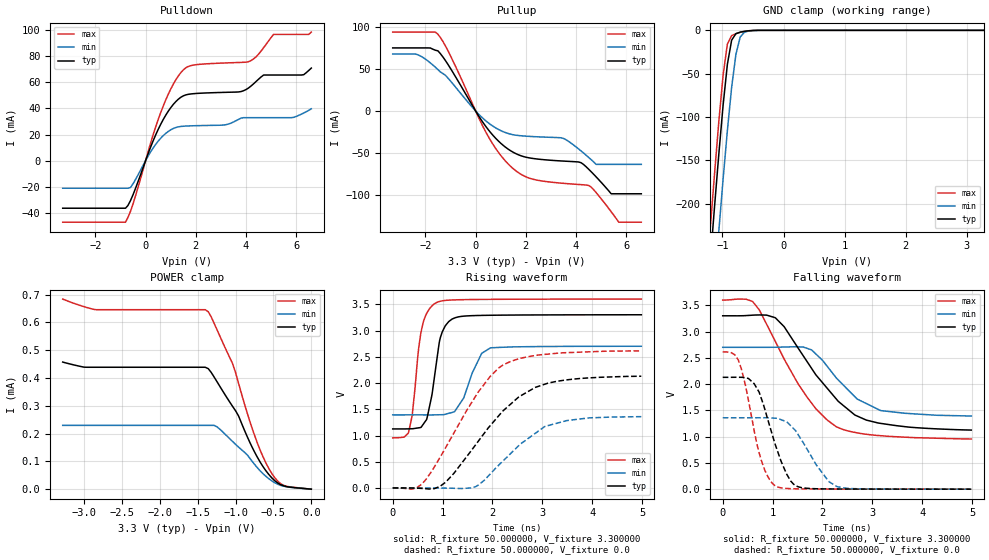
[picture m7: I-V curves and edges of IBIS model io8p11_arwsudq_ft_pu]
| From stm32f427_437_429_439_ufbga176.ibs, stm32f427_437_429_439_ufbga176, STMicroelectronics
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|   Model io8p11_arwsudq_ft_pu
[Model]  io8p11_arwsudq_ft_pu
Model_type I/O
Polarity   Non-Inverting
Enable   Active-Low
Vinl =   0.990000V
Vinh =   2.310000V
Vmeas =  1.650000V
Cref =   30.000000pF
Rref =   100.000000M
Vref =   0.0V
C_comp   2.905500pF   2.831700pF   2.987900pF
[Temperature Range]   25.000000   0.125000k   -40.000000
[Pullup Reference]   3.300000V   2.700000V   3.600000V
[Pulldown Reference]   0.0V   0.0V   0.0V
[POWER Clamp Reference]   3.300000V   2.700000V   3.600000V
[GND Clamp Reference]   0.0V   0.0V   0.0V
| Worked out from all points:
|   slope of the pulldown table from 0 to 0.495 V, typ, clamps not added: 20.9 ohm
|   slope of the pullup table from 0 to 0.495 V, typ, clamps not added: 22.6 ohm
|   GND clamp passes 1 mA (typ) near -0.62 V on its own axis
|   rising waveform, R_fixture 50.000000, V_fixture 3.300000: 20-80 % time 217ps typ, 339ps min, 190ps max; typ from 1.12 V to 3.3 V
|   rising waveform, R_fixture 50.000000, V_fixture 0.0: 20-80 % time 1.14ns typ, 965ps min, 1.02ns max; typ from 0.001 V to 2.13 V
|   falling waveform, R_fixture 50.000000, V_fixture 3.300000: 20-80 % time 1.07ns typ, 814ps min, 1ns max; typ from 3.3 V to 1.12 V
|   falling waveform, R_fixture 50.000000, V_fixture 0.0: 20-80 % time 436ps typ, 549ps min, 356ps max; typ from 2.13 V to 0.001 V
[Pulldown]
|Voltage   I(typ)   I(min)   I(max)
-3.3V     -36.39mA   -21.08mA   -47.09mA
-800mV    -36.39mA   -21.08mA   -47.09mA
-600mV    -30.5mA    -20.54mA   -38.69mA
700mV     31.4mA     19.11mA    41.71mA
1.2V      45.15mA    25.37mA    61.75mA
1.6V      50.35mA    26.5mA     71.06mA
3.1V      52.28mA    27.26mA    74.75mA
4.1V      55.65mA    32.92mA    75.79mA
4.7V      65.56mA    32.92mA    86.49mA
5.1V      65.56mA    32.92mA    96.69mA
6.3V      65.85mA    36.49mA    96.69mA
6.6V      70.9mA     39.7mA     98.44mA
[Pullup]
|Voltage   I(typ)   I(min)   I(max)
-3.3V     74.7mA     67.42mA    93.47mA
-2.3V     74.7mA     66.58mA    93.47mA
-1.5V     71.26mA    49mA       90.9mA
500mV     -22.06mA   -14mA      -30.02mA
1.6V      -50.64mA   -28.81mA   -70.96mA
3.5V      -59.52mA   -32.65mA   -85.91mA
4.2V      -61.44mA   -47.48mA   -87.45mA
4.5V      -69.08mA   -55.13mA   -88.39mA
4.8V      -78.23mA   -63.4mA    -96.87mA
5.4V      -98.3mA    -63.4mA    -119.6mA
5.7V      -98.3mA    -63.4mA    -132mA
6.6V      -98.3mA    -63.4mA    -132mA
[GND_clamp]
|Voltage   I(typ)   I(min)   I(max)
-3.3V     -2.317A    -2.396A    -2.29A
-1.2V     -266mA     -356.2mA   -228.4mA
-1.13V    -203.2mA   -293mA     -165.3mA
-1.06V    -142.7mA   -231.3mA   -105.2mA
-990mV    -86.51mA   -171.7mA   -51.78mA
-920mV    -39.3mA    -115.7mA   -15.93mA
-850mV    -11.37mA   -65.76mA   -6.097mA
-780mV    -3.83mA    -27.55mA   -3.88mA
-710mV    -2.09mA    -7.747mA   -2.382mA
-640mV    -1.147mA   -2.129mA   -1.22mA
-570mV    -523.9uA   -800uA     -476.9uA
3.28V     0A         0A         0A
[POWER_clamp]
|Voltage   I(typ)   I(min)   I(max)
-3.28V    457.2uA    229.4uA    683.8uA
-2.84V    438.5uA    229.4uA    645.6uA
-1.36V    433.5uA    229.4uA    638.5uA
-1.24V    384.6uA    223.2uA    570.8uA
-1.04V    298.3uA    171.8uA    452.6uA
-960mV    263.4uA    151.4uA    380.6uA
-760mV    139.5uA    92.81uA    202.3uA
-640mV    82.23uA    56.4uA     118uA
-560mV    52.51uA    37.37uA    73.96uA
-440mV    21.63uA    17.4uA     27.8uA
-360mV    11.48uA    10.27uA    13.1uA
0V        0A         0A         0A
[Ramp]
| variable   typ   min   max
dV/dt_r  1.26013/1.13320n   0.80385/0.95571n   1.56003/1.01363n
dV/dt_f  1.27506/1.05048n   0.76710/0.78758n   1.56877/0.99264n
R_load = 50.000000
[Rising Waveform]
R_fixture= 50.000000
V_fixture= 3.300000
V_fixture_min= 2.700000
V_fixture_max= 3.600000
|time   V(typ)   V(min)   V(max)
0s        1.125V     1.393V     955.6mV
320.3ps   1.127V     1.393V     1.069V
390.4ps   1.129V     1.393V     1.379V
570.6ps   1.159V     1.393V     2.981V
690.7ps   1.341V     1.393V     3.342V
860.9ps   2.279V     1.394V     3.523V
951ps     2.848V     1.396V     3.556V
1.121ns   3.168V     1.422V     3.578V
1.962ns   3.29V      2.67V      3.593V
4.985ns   3.3V       2.7V       3.599V
[Rising Waveform]
R_fixture= 50.000000
V_fixture= 0.0
V_fixture_min= 0.0
V_fixture_max= 0.0
|time   V(typ)   V(min)   V(max)
0s        1.438mV    1.24mV     1.772mV
480.5ps   -2.046mV   1.184mV    5.212mV
670.7ps   -14.12mV   1.224mV    168.5mV
961ps     40.14mV    -51.31uV   603.7mV
1.662ns   822.4mV    25.77mV    1.748V
2.202ns   1.461V     506.3mV    2.336V
2.533ns   1.738V     812.4mV    2.463V
3.053ns   1.979V     1.174V     2.545V
3.934ns   2.097V     1.336V     2.594V
4.985ns   2.129V     1.359V     2.612V
[Falling Waveform]
R_fixture= 50.000000
V_fixture= 3.300000
V_fixture_min= 2.700000
V_fixture_max= 3.600000
|time   V(typ)   V(min)   V(max)
0s        3.3V       2.7V       3.599V
600.6ps   3.312V     2.7V       3.57V
740.7ps   3.316V     2.7V       3.399V
1.051ns   3.264V     2.701V     2.819V
1.512ns   2.687V     2.708V     2.006V
1.782ns   2.3V       2.65V      1.639V
2.272ns   1.722V     2.124V     1.192V
2.653ns   1.411V     1.758V     1.08V
3.163ns   1.253V     1.498V     1.019V
4.985ns   1.125V     1.393V     955.6mV
[Falling Waveform]
R_fixture= 50.000000
V_fixture= 0.0
V_fixture_min= 0.0
V_fixture_max= 0.0
|time   V(typ)   V(min)   V(max)
0s        2.129V     1.359V     2.612V
310.3ps   2.13V      1.359V     2.464V
460.5ps   2.118V     1.359V     1.958V
630.6ps   2.008V     1.359V     1.117V
850.9ps   1.5V       1.361V     347.2mV
1.061ns   829.1mV    1.351V     61.22mV
1.421ns   95.78mV    1.153V     9.132mV
1.882ns   9.026mV    456.6mV    4.586mV
2.292ns   4.507mV    49.46mV    3.486mV
4.985ns   1.438mV    1.24mV     1.772mV
